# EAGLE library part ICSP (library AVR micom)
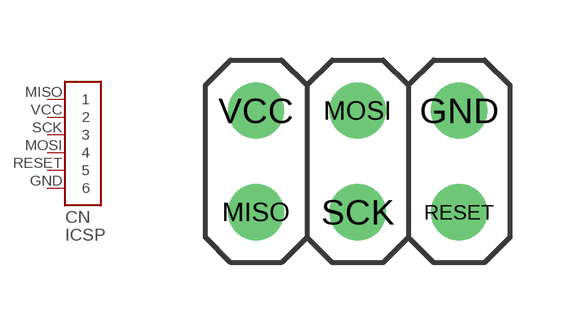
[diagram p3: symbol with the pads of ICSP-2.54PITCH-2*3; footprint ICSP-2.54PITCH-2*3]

Designator prefix CN

## ICSP2.54-2*3  [ICSP-2.54PITCH-2*3]
GND  6  pas
MISO  1  pas
MOSI  4  pas
RESET  5  pas
SCK  3  pas
VCC  2  pas

## Footprint ICSP-2.54PITCH-2*3 (pad centres in mm)
drill 0.9: GND 2.54,1.27; MISO -2.54,-1.27; MOSI 0,1.27; RESET 2.54,-1.27; SCK 0,-1.27; VCC -2.54,1.27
